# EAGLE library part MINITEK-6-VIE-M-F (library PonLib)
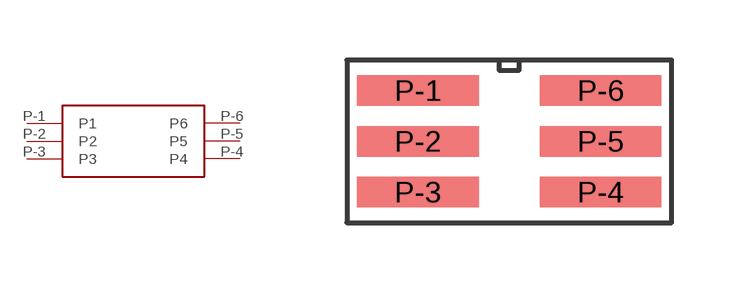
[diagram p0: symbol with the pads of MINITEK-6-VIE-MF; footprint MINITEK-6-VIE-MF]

Designator prefix -

## MINITEK-6-VIE-M-F  [MINITEK-6-VIE-MF]
P-1  P1
P-2  P2
P-3  P3
P-4  P4
P-5  P5
P-6  P6

## Footprint MINITEK-6-VIE-MF (pad centres in mm)
smd 3.048 x 0.762: P-1 -2.286,1.27; P-2 -2.286,0; P-3 -2.286,-1.27; P-4 2.286,-1.27; P-5 2.286,0; P-6 2.286,1.27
